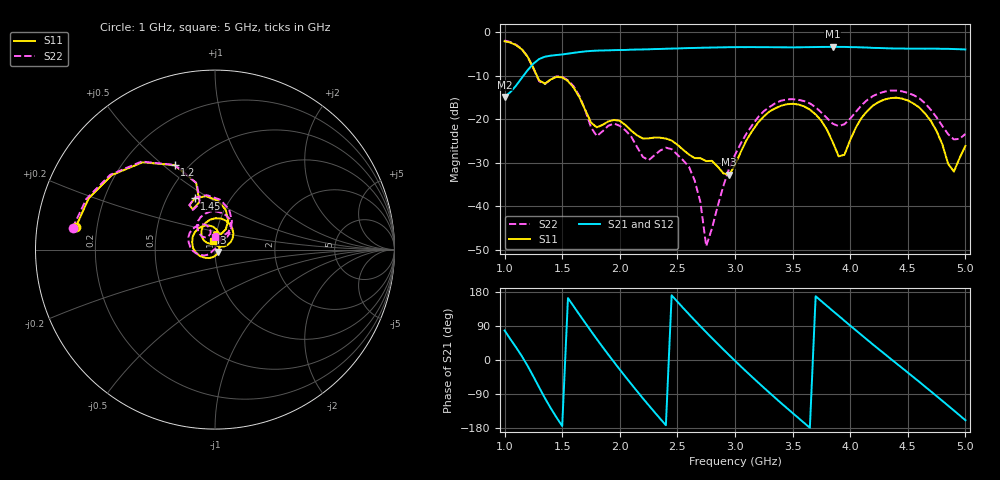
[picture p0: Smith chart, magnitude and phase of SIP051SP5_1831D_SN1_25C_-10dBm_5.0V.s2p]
# GHz  S  dB  R  50
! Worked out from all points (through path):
!   81 points, 1 GHz to 5 GHz, reference 50 ohm
!   highest |S21| = -3.37 dB at 3.85 GHz (marker M1); lowest = -14.9 dB at 1 GHz (marker M2)
!   lowest |S11| = -32.7 dB at 2.95 GHz (marker M3), VSWR 1.05, Z = 51.9 - j1.39 ohm
!   |S11| at or under -10 dB: 1.281 GHz to end of sweep
!   |S22| runs from -49.2 to -1.9 dB; largest |S21 - S12| = 0.0029
!   S11 on the Smith chart (normalised r, x): 1 GHz: 0.12, +0.08; 1.2 GHz: 0.42, +0.55; 1.45 GHz: 0.69, +0.43; 5 GHz: 0.97, +0.09
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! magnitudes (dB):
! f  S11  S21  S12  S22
! 1 GHz  -2.1  -14.9  -14.9  -1.9
! 1.2 GHz  -5.7  -8.7  -8.7  -5.6
! 1.3 GHz  -11.1  -6.2  -6.2  -11.3
! 1.45 GHz  -10.3  -5.3  -5.2  -10.1
! 1.7 GHz  -17.9  -4.4  -4.4  -17.9
! 1.8 GHz  -21.9  -4.2  -4.2  -23.9
! 1.95 GHz  -20.2  -4.1  -4.1  -21.0
! 2.2 GHz  -24.4  -4.0  -4.0  -28.7
! 2.35 GHz  -24.3  -3.9  -3.9  -27.2
! 2.6 GHz  -28.1  -3.7  -3.7  -30.9
! 2.7 GHz  -29.0  -3.6  -3.6  -39.1
! 2.75 GHz  -29.6  -3.6  -3.6  -49.2
! 2.95 GHz  -32.7  -3.5  -3.5  -31.2
! 3 GHz  -30.6  -3.4  -3.4  -28.2
! 3.3 GHz  -18.2  -3.5  -3.5  -17.2
! 3.7 GHz  -18.9  -3.4  -3.4  -17.3
! 3.85 GHz  -25.4  -3.4  -3.4  -21.0
! 3.95 GHz  -28.2  -3.4  -3.4  -21.2
! 4.35 GHz  -15.2  -3.7  -3.7  -13.4
! 4.65 GHz  -18.7  -3.8  -3.8  -16.3
! 4.9 GHz  -32.0  -3.9  -3.9  -24.6
! 5 GHz  -26.1  -4.0  -4.0  -23.4
